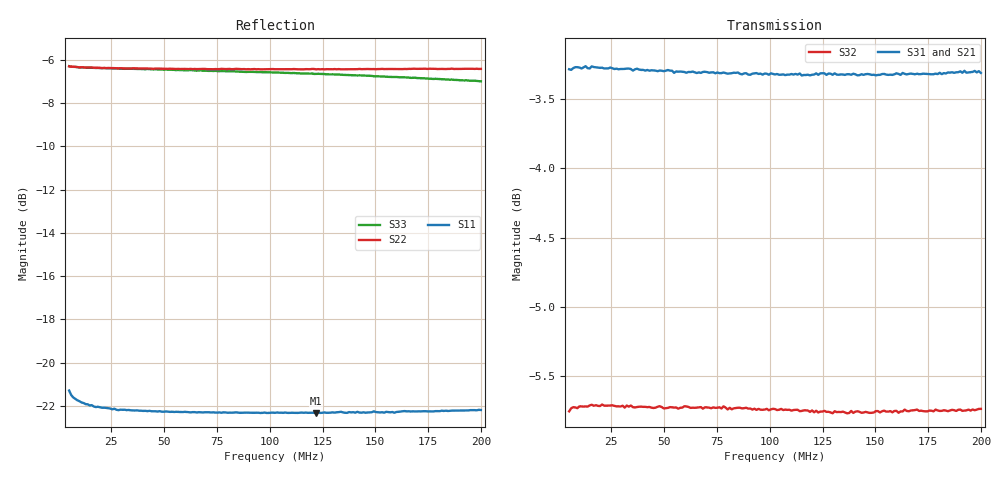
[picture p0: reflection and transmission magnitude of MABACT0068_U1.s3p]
#	MHz	S	RI	R	75
!FREQ	R1	I1	R2	I2	R3	I3
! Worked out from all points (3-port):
!   201 points, 5 MHz to 200 MHz, reference 75 ohm
!   strongest paths, dB at 5 MHz, 53.75 MHz, 102.5 MHz, 151.2 MHz, 200 MHz:
!     S31: -3.3, -3.3, -3.3, -3.3, -3.3
!     S21: -3.3, -3.3, -3.4, -3.5, -3.6
!     S32: -5.8, -5.7, -5.7, -5.8, -5.7
!   lowest |S11| = -22.3 dB at 122 MHz (marker M1), VSWR 1.17, Z = 64.5 + j1.88 ohm
!   |S11| at or under -10 dB: start of sweep to end of sweep
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5  -0.0844 0.018  0.6849 0.00397  -0.6854 -0.00467
   0.6847 0.00394  -0.4836 0.0136  -0.5134 -0.00497
   -0.6854 -0.00467  -0.5153 -0.00531  -0.484 0.0136
6.95  -0.0819 0.0149  0.686 -0.0015  -0.686 0.00198
      0.6863 -0.00162  -0.4827 0.0131  -0.5139 -0.0014
      -0.686 0.00198  -0.5172 -0.0014  -0.4822 0.0132
12.8  -0.0797 0.00982  0.6867 -0.0141  -0.687 0.0144
      0.6862 -0.0132  -0.4802 0.0136  -0.5153 0.00613
      -0.687 0.0144  -0.5175 0.00543  -0.4803 0.0146
28.4  -0.0773 0.00793  0.6843 -0.0377  -0.6843 0.0387
      0.6851 -0.037  -0.4782 0.0215  -0.5143 0.0193
      -0.6843 0.0387  -0.5172 0.0192  -0.4776 0.0226
72.275  -0.0761 0.00994  0.6744 -0.0976  -0.6761 0.1006
        0.6748 -0.0983  -0.4741 0.0473  -0.5118 0.0535
        -0.6761 0.1006  -0.5139 0.053  -0.4697 0.0495
102.5  -0.0756 0.0127  0.663 -0.136  -0.6676 0.1412
       0.664 -0.137  -0.4719 0.0653  -0.5084 0.0749
       -0.6676 0.1412  -0.5107 0.0757  -0.463 0.0674
122  -0.0751 0.0145  0.6554 -0.1609  -0.6625 0.1662
     0.6552 -0.1616  -0.4697 0.0773  -0.5056 0.089
     -0.6625 0.1662  -0.5078 0.0896  -0.4582 0.0782
133.7  -0.0754 0.0159  0.6496 -0.1752  -0.658 0.1812
       0.6494 -0.1761  -0.4685 0.085  -0.5038 0.0968
       -0.658 0.1812  -0.5057 0.0974  -0.4549 0.0849
168.8  -0.0745 0.0203  0.6306 -0.2179  -0.6438 0.2265
       0.6314 -0.218  -0.4655 0.1067  -0.4981 0.1214
       -0.6438 0.2265  -0.5013 0.122  -0.4435 0.103
200  -0.0737 0.025  0.6115 -0.2541  -0.6292 0.2663
     0.6109 -0.2555  -0.46 0.1271  -0.4934 0.1436
     -0.6292 0.2663  -0.4958 0.1443  -0.4308 0.119
